(* Logix 5000 AddOnInstructionDefinition export; software revision 16.00 *)

ADD_ON_INSTRUCTION AMCI_ANG1E_Clear_driver_fault   (* revision 1.0, vendor AMCI *)
VAR_IN_OUT
   AMCI_ANG1E_output_data : INT[10]; {required}
END_VAR
VAR
   command_data_block : INT[10];
        [0]   // Command Bits MSW
        [1]   // Command Bits LSW
        [2]   // Upper Target Position
        [3]   // Lower Target Position
        [4]   // Upper Programmed Speed
        [5]   // Lower Programmed Speed
END_VAR

ROUTINE Logic   (* ladder *)
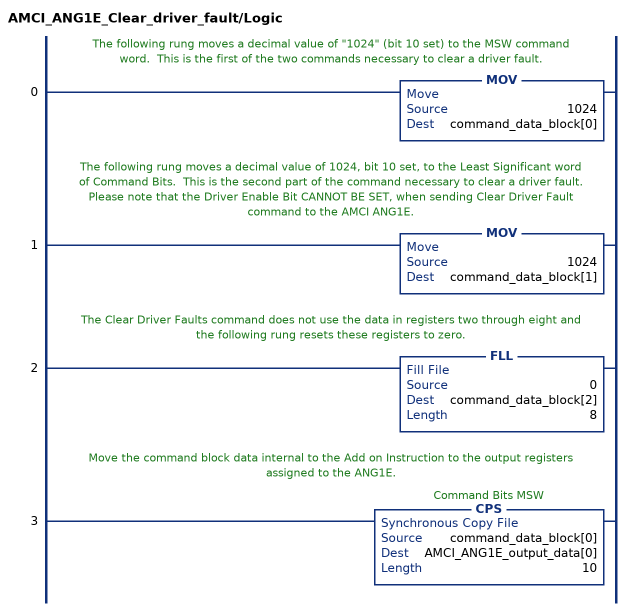
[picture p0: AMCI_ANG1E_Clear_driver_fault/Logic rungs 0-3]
   // The following rung moves a decimal value of "1024" (bit 10 set) to the MSW command word.  This is the first of the two commands necessary to clear a driver fault.
   0: MOV(1024,command_data_block[0]);
   // The following rung moves a decimal value of 1024, bit 10 set, to the Least Significant word of Command Bits.  This is the second part of the command necessary to clear a driver fault.
   // Please note that the Driver Enable Bit CANNOT BE SET, when sending Clear Driver Fault command to the AMCI ANG1E.
   1: MOV(1024,command_data_block[1]);
   // The Clear Driver Faults command does not use the data in registers two through eight and the following rung resets these registers to zero.
   2: FLL(0,command_data_block[2],8);
   // Move the command block data internal to the Add on Instruction to the output registers assigned to the ANG1E.
   3: CPS(command_data_block[0],AMCI_ANG1E_output_data[0],10);
END_ROUTINE
END_ADD_ON_INSTRUCTION
